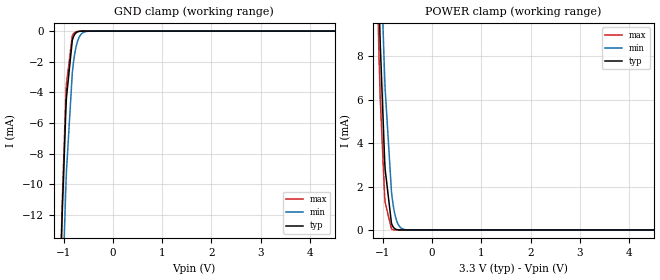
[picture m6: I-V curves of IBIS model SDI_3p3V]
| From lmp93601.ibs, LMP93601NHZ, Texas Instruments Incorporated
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|   Model SDI_3p3V
[Model]   SDI_3p3V
Model_type   Input
Vinl = .9
Vinh = 2.52
|   typ   min   max
|   (nom PVT)   (fast PVT)   (slow PVT)
C_comp   0.1436pF   0.1360pF   0.1525pF
[Model spec]
|subparameter
Vinl   0.99   0.9   1.08
Vinh   2.31   2.1   2.52
[Voltage Range]   3.3   3.0   3.6
[Temperature Range]   27   125   -25
[Power Clamp Reference]   3.3   3.0   3.6
[GND Clamp Reference]   0   0   0
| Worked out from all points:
|   GND clamp passes 1 mA (typ) near -0.84 V on its own axis
|   POWER clamp passes 1 mA (typ) near -0.86 V on its own axis
[GND Clamp]
|   Voltage   I(typ)   I(min)   I(max)
-3.3V     -526.6mA   -475.1mA   -563.8mA
-1.053V   -14.66mA   -20.34mA   -14.17mA
-1.043V   -13.41mA   -19.13mA   -12.81mA
-1.033V   -12.21mA   -17.95mA   -11.52mA
-953.7mV  -4.958mA   -9.976mA   -4.047mA
-943.8mV  -4.34mA    -9.17mA    -3.458mA
-825mV    -605.9uA   -2.736mA   -319.1uA
-785.4mV  -264.9uA   -1.684mA   -117.1uA
-745.8mV  -104.2uA   -992.6uA   -37.98uA
-646.8mV  -6.219uA   -211.1uA   -1.128uA
-468.6mV  -9.255nA   -4.518uA   0A
6.59V     0A         0A         0A
[POWER Clamp]
|   Voltage   I(typ)   I(min)   I(max)
-3.3V     323.2mA    295.8mA    340.5mA
-1.181V   20.82mA    24.71mA    18.6mA
-1.082V   10.98mA    15.56mA    8.388mA
-1.063V   9.324mA    13.92mA    6.763mA
-1.053V   8.542mA    13.13mA    6.018mA
-963.6mV  3.189mA    7.041mA    1.538mA
-953.7mV  2.79mA     6.49mA     1.273mA
-825mV    302.4uA    1.756mA    45.52uA
-805.2mV  195.7uA    1.376mA    22.75uA
-696.3mV  9.709uA    289.4uA    255.6nA
-528mV    22.12nA    9.496uA    0A
6.59V     0A         0A         0A
